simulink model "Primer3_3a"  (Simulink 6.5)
settings: Solver=ode23t  SolverMode=SingleTasking  StartTime=0.0  StopTime=1  RelTol=1e-3  AbsTol=1e-6
undefined symbols (not defined in the file or in its folder): Continuous, powergui, steady, ZData
libraries: powerlib x4, powerlib_extras x1

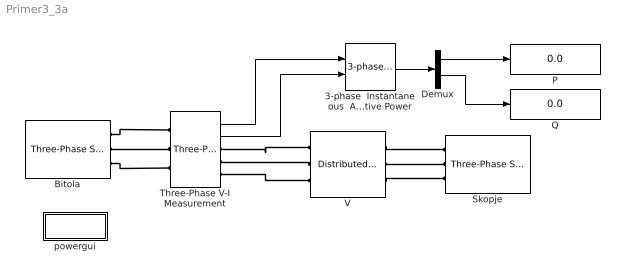
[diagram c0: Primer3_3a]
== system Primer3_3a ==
  3-phase  Instantaneous  Active & Reactive Power : powerlib_extras/Measurements/3-phase  Instantaneous  Active & Reactive Power  DialogController=PMDialogs.PMDefaultMaskDlg  SystemSampleTime=-1
  Bitola : powerlib/Electrical Sources/Three-Phase Source  DialogController=PMDialogs.PMDefaultMaskDlg  SystemSampleTime=-1  Voltage=410e3  PhaseAngle=0  Frequency=50  InternalConnection=Yg  SpecifyImpedance=on  Resistance=0.8929  Inductance=16.58e-3  ShortCircuitLevel=sqrt(3)*400e3*16e3  BaseVoltage=400e3  XRratio=10
  Demux : Demux  Outputs=2
  P : Display
  Q : Display
  Skopje : powerlib/Electrical Sources/Three-Phase Source  Orientation=left  DialogController=PMDialogs.PMDefaultMaskDlg  SystemSampleTime=-1  Voltage=395e3  PhaseAngle=-2.5  Frequency=50  InternalConnection=Yg  SpecifyImpedance=on  Resistance=0.8929  Inductance=16.58e-3  ShortCircuitLevel=sqrt(3)*400e3*14e3  BaseVoltage=400e3  XRratio=10
  Three-Phase V-I Measurement : powerlib/Measurements/Three-Phase V-I Measurement  DialogController=PMDialogs.PMDefaultMaskDlg  SystemSampleTime=-1  VoltageMeasurement=phase-to-ground  SetLabelV=off  LabelV=Vabc  Vpu=off  CurrentMeasurement=yes  SetLabelI=off  LabelI=Iabc  Ipu=off  Pbase=100e6  Vbase=500e3  OutputType=Complex  PhasorSimulation=off  PSBequivalent=0
  V : powerlib/Elements/Distributed Parameters Line  DialogController=PMDialogs.PMDefaultMaskDlg  SystemSampleTime=-1  Phases=3  Frequency=50  Resistance=[0.029983 0.29405]  Inductance=[0.0010055 0.0025377]  Capacitance=[1.1784e-008 8.6541e-009]  Length=113.5  x1=[0 8.60953493752654e-011 155617.901806502 -377100.173822709;0.000106379256748321 8.65325079837872e-011 168131.358149619 -371689.815392539;0.000212758513496643 8.68730275722288e-011 180457.046333984 -365864.355859094;0.000319137770244964 8.7116527850222e-011 192581.201100092 -359630.30106294;0.000425517026993286 8.72627368780204e-011 204490.282259832 -352994.613161546;0.000531896283741607 8.7311491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  x2=[0 1.52828084545043e-010 143893.096531519 -373225.666404169;0.000106379256748321 1.57548911798779e-010 156283.637924653 -368209.241884694;0.000212758513496643 1.62093789310554e-010 168499.6426266 -362781.603346936;0.000319137770244964 1.66457641386629e-010 180527.467871754 -356948.812347202;0.000425517026993286 1.70635594501455e-010 192353.681052273 -350717.382913801;0.000531896283741607 1.7462298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  x3=[0 -7.90373299703389e-013 525.422105317868 -979.122392884629;0.000106379256748321 -7.55164225839465e-013 557.844919090553 -961.019300144194;0.000212758513496643 -7.19111788799262e-013 589.644734783168 -941.842946433889;0.000319137770244964 -6.82256251742466e-013 620.786038539719 -921.614747798094;0.000425517026993286 -6.44638774726363e-013 651.234051926655 -900.357294975707;0.000531896283741607 -6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  x4=[0 1.19047082254412e-012 334.073009196058 -1629.8040871509;0.000106379256748321 1.13114510037133e-012 388.344425208523 -1617.73135760439;0.000212758513496643 1.07055612168819e-012 442.182140342785 -1603.85195474176;0.000319137770244964 1.0087715519266e-012 495.52602894023 -1588.18137900235;0.000425517026993286 9.45860391747901e-013 548.316516844957 -1570.73713119736;0.000531896283741607 8.81892899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  x5=0.000531896283741607  Measurements=None
  powergui : Subsystem  AncestorBlock=powerlib/powergui  InitFcn=powergui( 'InitFcn_Callback' , gcb , 0 , [ ] );  mask(PSB option menu block){SimulationMode=Continuous, SampleTime=50e-6, echomessages=off, RestoreLinks=warning, x0status=steady, Frange=[0:2:500], Ylog=off, Xlog=on, ShowGrid=off, save=off, variable=ZData, structure=, ZoomFFT=on, StartTime=0.0, cycles=1, DisplayStyle=1, fundamental=60, FreqAxis=off, MaxFrequency=1000, frequencyindice=50, frequencyindicesteady=1, RmsSteady=2, display=off, Ts=0, frequency=60, methode=off, HookPort=off, Interpol=off}
      mask prompts: SimulationMode "Simulation mode"; SampleTime "Sample time Ts (when simulation mode is Discrete) (s)"; echomessages "Echo  Messages"; RestoreLinks "Restore disabled links"; x0status "Initial electrical states status"; Frange "Impedance tool: Frequency Range"; Ylog "Impedance tool: Log impedance"; Xlog "Impedance tool: log Frequency"; ShowGrid "Impedance tool: grid"; save "Impedance tool: Save Data To Workspace"; variable "Impedance tool: Variable Name"; structure "Structure Name (PSBFFTSCOPE)"; ZoomFFT "ZoomFFT (PSBFFTSCOPE)"; StartTime "Start Time (PSBFFTSCOPE)"; cycles "Cycles (PSBFFTSCOPE)"; DisplayStyle "Display style (PSBFFTSCOPE)"; fundamental "Fundamental (PSBFFTSCOPE)"; FreqAxis "Frequency Axis (PSBFFTSCOPE)"; MaxFrequency "Max Frequency (PSBFFTSCOPE)"; frequencyindice "Load flow frequency (Hz)"; frequencyindicesteady "Frequency indice (STEADYSTATE)"; RmsSteady "RMS display (STEADYSTATE)"; display "Display Results"; Ts "OBSOLETE 1"; frequency "Phasor frequency (Hz)"; methode "Phasor simulation"; HookPort "Hook port"; Interpol "Interpolate"
      mask init:
      | powerlibroot = which('powersysdomain');
      | PSBroot = powerlibroot(1:end-16);
      | %
      | switch SimulationMode
      | 	case 1
      | 		message=sprintf('Continuous');
      | 	case 2
      |         SampleTimeeval=evalin('base',SampleTime,'NaN');
      |         if isnan(SampleTimeeval)
      |             message=sprintf('Warning !!,\nUndefined sample time');
      |         else
      |             message=sprintf('Discrete,\nTs = %.4g s.',SampleTimeeval);
      |         end
      | 	case 3
      | 		message=sprintf('Phasors');
      | end
      | if strcmp(bdroot,'powerlib')
      |   message='powergui';
      | end
      | power_initmask();
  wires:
  Three-Phase V-I Measurement/1 -> 3-phase  Instantaneous  Active & Reactive Power/1
  Three-Phase V-I Measurement/2 -> 3-phase  Instantaneous  Active & Reactive Power/2
  3-phase  Instantaneous  Active & Reactive Power/1 -> Demux/1
  Demux/1 -> P/1
  Demux/2 -> Q/1
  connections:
  Bitola/RConn1 -- Three-Phase V-I Measurement/LConn1
  Bitola/RConn2 -- Three-Phase V-I Measurement/LConn2
  Bitola/RConn3 -- Three-Phase V-I Measurement/LConn3
  V/RConn1 -- Skopje/RConn1
  V/RConn2 -- Skopje/RConn2
  V/RConn3 -- Skopje/RConn3
  V/LConn2 -- Three-Phase V-I Measurement/RConn2
  V/LConn1 -- Three-Phase V-I Measurement/RConn1
  V/LConn3 -- Three-Phase V-I Measurement/RConn3

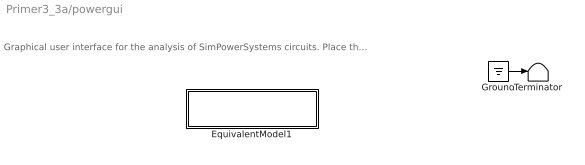
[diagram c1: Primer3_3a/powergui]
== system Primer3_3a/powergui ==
  note: Graphical user interface for the analysis of SimPowerSystems circuits. Place the Powergui block in the top-level of your model and double-click on it to open the GUI.
  EquivalentModel1 : Subsystem
  Ground : Ground
  Terminator : Terminator
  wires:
  Ground/1 -> Terminator/1

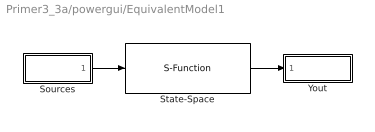
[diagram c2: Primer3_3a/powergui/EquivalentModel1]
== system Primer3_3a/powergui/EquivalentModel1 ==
  Sources : Subsystem
  State-Space : S-Function  FunctionName=sfun_spssw_contc  Parameters=A, B, C, D, x0
  Yout : Subsystem
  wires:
  State-Space/1 -> Yout/1(v,i)
  Sources/1(u) -> State-Space/1

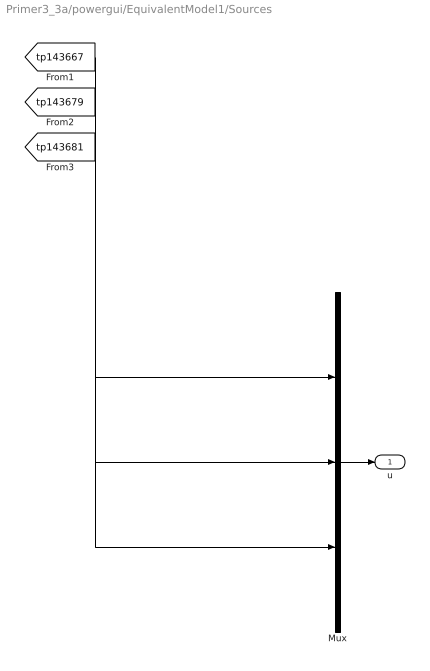
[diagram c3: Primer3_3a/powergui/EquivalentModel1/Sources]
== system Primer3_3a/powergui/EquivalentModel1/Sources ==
  Mux : Mux  Inputs=[6 3 3]
  u : Outport
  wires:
  Mux/1 -> u/1
  [tp143667] -> Mux/1
  [tp143679] -> Mux/2
  [tp143681] -> Mux/3

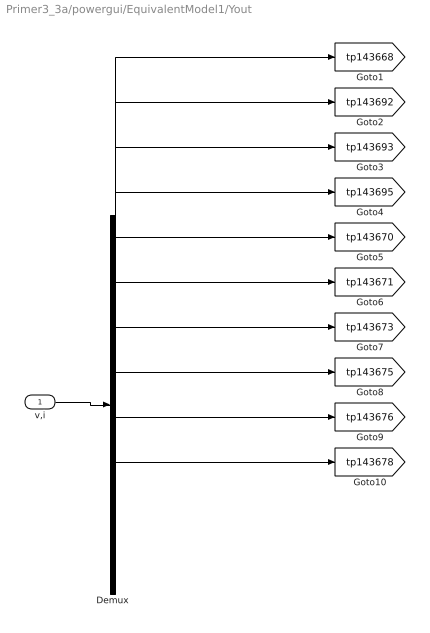
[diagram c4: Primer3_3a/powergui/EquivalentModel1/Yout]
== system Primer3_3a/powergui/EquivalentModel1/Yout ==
  v,i : Inport
  Demux : Demux  Outputs=[6 1 1 1 1 1 1 1 1 1]
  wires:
  v,i/1 -> Demux/1
  Demux/1 -> [tp143668]
  Demux/2 -> [tp143692]
  Demux/3 -> [tp143693]
  Demux/4 -> [tp143695]
  Demux/5 -> [tp143670]
  Demux/6 -> [tp143671]
  Demux/7 -> [tp143673]
  Demux/8 -> [tp143675]
  Demux/9 -> [tp143676]
  Demux/10 -> [tp143678]
